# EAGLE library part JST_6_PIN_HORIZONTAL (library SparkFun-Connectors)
JST 6 pin horizontal connector JST-SH type. Here is the connector we sell at SparkFun: name (XXX-00000) Datasheet It was used on these SparkFun products: name (XXX-00000) name (XXX-00000)
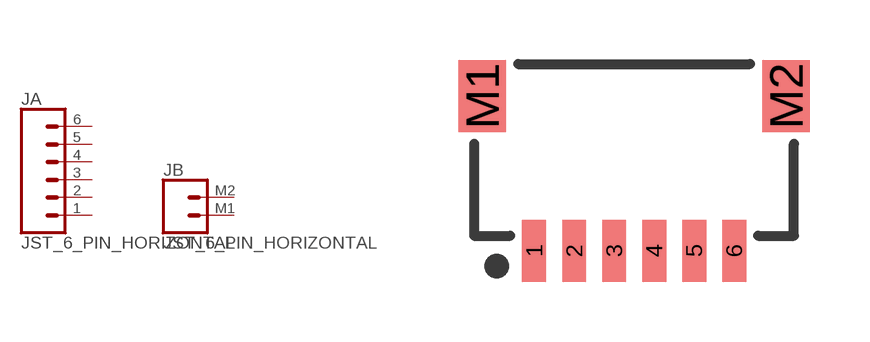
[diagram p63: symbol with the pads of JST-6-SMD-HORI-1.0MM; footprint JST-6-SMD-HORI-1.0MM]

Designator prefix J; gates A=CONN_06 B=CONN_02

## JST_6_PIN_HORIZONTAL (PROD_ID: XXX-00000; VALUE: BM06B-SRSS-TB)  [JST-6-SMD-HORI-1.0MM]
1  A:1  pas
2  A:2  pas
3  A:3  pas
4  A:4  pas
5  A:5  pas
6  A:6  pas
M1  B:1  pas
M2  B:2  pas

## Footprint JST-6-SMD-HORI-1.0MM (pad centres in mm)
JST SH Vertical 6-Pin SMT Specifications: Pin count:6 Pin pitch: 1 mm Datasheet referenced for footprint Example device(s): JST_6PIN_VERTICAL
smd 0.6 x 1.55: 1 -2.5,-4.775; 2 -1.5,-4.775; 3 -0.5,-4.775; 4 0.5,-4.775; 5 1.5,-4.775; 6 2.5,-4.775
smd 1.2 x 1.8: M1 -3.8,-0.9; M2 3.8,-0.9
